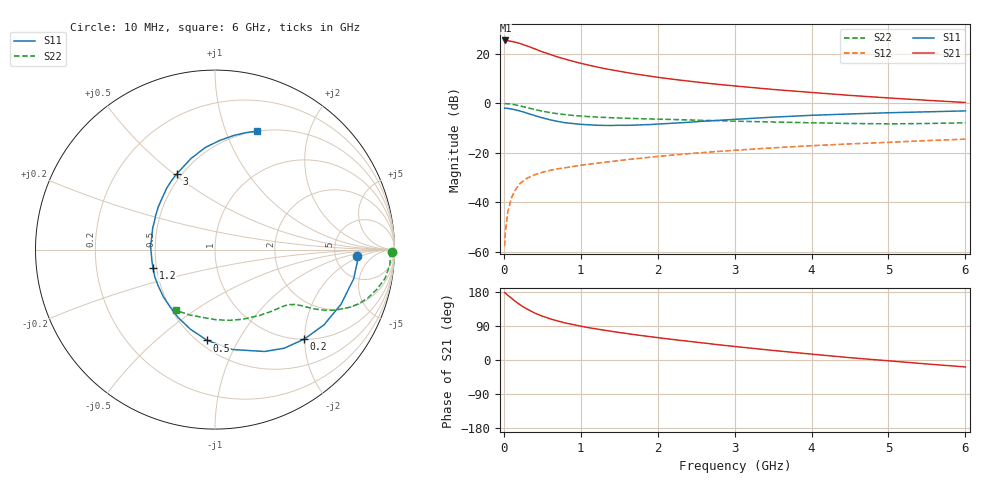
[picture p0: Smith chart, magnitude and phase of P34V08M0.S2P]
! SIEMENS Small Signal Semiconductors
! BFP181
! Si NPN RF Bipolar Junction Transistor in SOT143
! VCE = 4 V  IC = 8 mA
! Common Emitter S-Parameters:  March  1996
# GHz  S  MA  R  50
!  f  S11  S21  S12  S22
! GHz  MAG  ANG  MAG  ANG  MAG  ANG  MAG  ANG
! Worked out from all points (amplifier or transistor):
!   36 points, 10 MHz to 6 GHz, reference 50 ohm
!   highest |S21| = 25.4 dB at 20 MHz (marker M1)
!   |S21| within 3 dB of that: start of sweep to 369 MHz
!   unconditionally stable (mu >= 1): 1.35 GHz to end of sweep
!   at 250 MHz: K = 0.28, MSG = 27.6 dB, |S12| = -31.4 dB
!   at 1.4 GHz: K = 1.01, MAG = 17.8 dB, |S12| = -23.5 dB
!   at 6 GHz: K = 1.01, MAG = 6.7 dB, |S12| = -14.5 dB
!   S11 on the Smith chart (normalised r, x): 10 MHz: 8.39, -1.50; 200 MHz: 1.01, -1.99; 500 MHz: 0.55, -0.75; 1.2 GHz: 0.48, -0.11; 3 GHz: 0.47, +0.51; 6 GHz: 0.50, +1.30
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0.01  0.7931 -2.4  18.49 177.9  0.0013 82.8  0.9848 -0.8
0.02  0.7962 -4.7  18.56 176.6  0.0025 86.1  0.9785 -1.8
0.05  0.7896 -11.9  18.34 171.1  0.0063 88.4  0.9778 -4.9
0.1  0.7652 -23.5  17.72 162.8  0.0124 76.2  0.9612 -9.6
0.15  0.7378 -34.7  17.12 154.5  0.0178 73.0  0.9282 -13.8
0.2  0.704 -45.1  16.33 147.2  0.0231 68.1  0.8939 -17.5
0.25  0.6714 -54.9  15.33 140.4  0.0268 64.0  0.8565 -20.6
0.3  0.6316 -64.0  14.43 134.7  0.0305 61.2  0.8175 -23.1
0.4  0.5654 -80.0  12.6 124.0  0.036 55.5  0.7492 -26.8
0.5  0.5077 -94.9  10.95 115.6  0.0403 52.1  0.6935 -29.1
0.6  0.464 -107.3  9.729 108.8  0.0442 49.9  0.6484 -30.7
0.7  0.4305 -118.5  8.588 102.9  0.0474 48.5  0.6145 -31.7
0.8  0.4037 -128.8  7.778 97.7  0.0499 47.7  0.5887 -32.5
1.1  0.3682 -155.8  5.915 85.3  0.0587 46.3  0.5382 -34.6
1.2  0.3603 -163.4  5.448 82.1  0.0613 45.8  0.5277 -35.5
1.7  0.3616 165.8  3.925 66.9  0.0757 45.3  0.4921 -40.2
2.2  0.3957 143.0  3.053 54.0  0.0901 43.6  0.4694 -46.4
3  0.4733 116.6  2.24 35.7  0.1122 39.2  0.4349 -58.6
3.5  0.5246 104.8  1.902 25.2  0.1259 36.0  0.4188 -67.7
4.5  0.6082 87.6  1.443 6.1  0.1511 28.6  0.3912 -88.9
5.5  0.6718 75.6  1.149 -10.5  0.1764 21.8  0.3905 -111.4
6  0.7016 70.3  1.037 -18.3  0.1884 17.9  0.4028 -122.8
